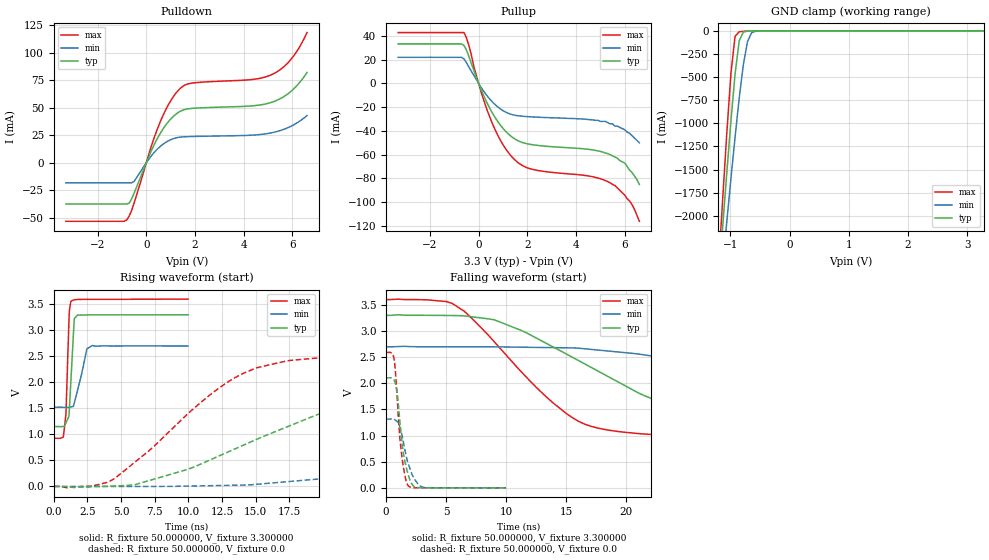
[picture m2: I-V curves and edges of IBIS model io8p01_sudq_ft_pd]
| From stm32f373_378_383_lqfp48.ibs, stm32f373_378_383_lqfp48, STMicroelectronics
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|   Model io8p01_sudq_ft_pd
[Model]  io8p01_sudq_ft_pd
Model_type I/O
Polarity   Non-Inverting
Enable   Active-Low
Vinl =   0.990000V
Vinh =   2.310000V
Vmeas =  1.650000V
Cref =   50.000000pF
Rref =   100.000000M
Vref =   0.0V
C_comp   1.970900pF   1.892300pF   2.063200pF
[Temperature Range]   25.000000   0.125000k   -40.000000
[Pullup Reference]   3.300000V   2.700000V   3.600000V
[Pulldown Reference]   0.0V   0.0V   0.0V
[POWER Clamp Reference]   3.300000V   2.700000V   3.600000V
[GND Clamp Reference]   0.0V   0.0V   0.0V
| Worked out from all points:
|   slope of the pulldown table from 0 to 0.495 V, typ, clamps not added: 20.9 ohm
|   slope of the pullup table from 0 to 0.495 V, typ, clamps not added: 22.2 ohm
|   GND clamp passes 1 mA (typ) near -0.64 V on its own axis
|   rising waveform, R_fixture 50.000000, V_fixture 3.300000: 20-80 % time 269ps typ, 640ps min, 200ps max; typ from 1.15 V to 3.3 V
|   rising waveform, R_fixture 50.000000, V_fixture 0.0: 20-80 % time 12.6ns typ, 30.4ns min, 7.07ns max; typ from 0 V to 2.1 V
|   falling waveform, R_fixture 50.000000, V_fixture 3.300000: 20-80 % time 11ns typ, 22.7ns min, 6.9ns max; typ from 3.3 V to 1.15 V
|   falling waveform, R_fixture 50.000000, V_fixture 0.0: 20-80 % time 664ps typ, 860ps min, 541ps max; typ from 2.1 V to 0 V
[Pulldown]
|Voltage   I(typ)   I(min)   I(max)
-3.3V     -37.45mA   -18.2mA    -53.24mA
-800mV    -37.45mA   -18.2mA    -51.9mA
-700mV    -36.7mA    -18.2mA    -48.48mA
-500mV    -27.71mA   -17.01mA   -36.66mA
200mV     10.57mA    6.084mA    14.57mA
500mV     23.91mA    13.38mA    33.24mA
900mV     37.17mA    19.88mA    52.48mA
1.3V      45.55mA    23.01mA    65.5mA
1.8V      49.29mA    23.83mA    72.18mA
5.1V      54.68mA    27.07mA    79.72mA
5.9V      64.2mA     32.82mA    93.01mA
6.6V      82.13mA    42.97mA    118.5mA
[Pullup]
|Voltage   I(typ)   I(min)   I(max)
-3.3V     33.17mA    21.9mA     42.7mA
-600mV    31.87mA    20.58mA    42.7mA
-400mV    22.79mA    13.76mA    31.9mA
100mV     -5.13mA    -3.299mA   -6.952mA
500mV     -22.5mA    -14.16mA   -30.52mA
900mV     -35.28mA   -21.55mA   -48mA
1.4V      -45.55mA   -26.41mA   -62.54mA
2.2V      -51.57mA   -28.22mA   -72.25mA
5.3V      -59.1mA    -33mA      -82.6mA
6V        -67mA      -39mA      -94mA
6.2V      -73mA      -42mA      -99mA
6.6V      -85mA      -50mA      -116mA
[GND_clamp]
|Voltage   I(typ)   I(min)   I(max)
-3.3V     -9.525A    -9.501A    -9.513A
-1.2V     -2.719A    -3.023A    -2.568A
-1.13V    -2.122A    -2.541A    -1.826A
-1.06V    -1.537A    -2.065A    -1.111A
-990mV    -975.7mA   -1.599A    -462mA
-920mV    -467.5mA   -1.149A    -59.02mA
-850mV    -106.6mA   -727.3mA   -10.13mA
-780mV    -13.08mA   -365.4mA   -5.271mA
-710mV    -3.06mA    -114.8mA   -2.651mA
-640mV    -957.2uA   -20.17mA   -921.6uA
-570mV    -212.9uA   -3.969mA   -172uA
3.28V     83.81uA    63.75uA    93.54uA
[POWER_clamp]
|Voltage   I(typ)   I(min)   I(max)
-3.28V    0A         0A         0A
0V        0A         0A         0A
[Ramp]
| variable   typ   min   max
dV/dt_r  1.26156/12.54362n   0.78870/30.38144n   1.55370/7.05539n
dV/dt_f  1.28928/10.94568n   0.70680/22.67171n   1.60430/6.89156n
R_load = 50.000000
[Rising Waveform]
R_fixture= 50.000000
V_fixture= 3.300000
V_fixture_min= 2.700000
V_fixture_max= 3.600000
|time   V(typ)   V(min)   V(max)
0s        1.15V      1.52V      925.1mV
720.7ps   1.152V     1.52V      978.8mV
900.9ps   1.221V     1.519V     1.392V
1.141ns   1.421V     1.522V     3.31V
1.261ns   1.999V     1.527V     3.552V
1.522ns   3.227V     1.604V     3.586V
1.762ns   3.293V     1.85V      3.592V
2.462ns   3.296V     2.645V     3.594V
2.863ns   3.297V     2.708V     3.595V
9.97ns    3.299V     2.699V     3.599V
[Rising Waveform]
R_fixture= 50.000000
V_fixture= 0.0
V_fixture_min= 0.0
V_fixture_max= 0.0
|time   V(typ)   V(min)   V(max)
0s        1.98nV     11.35nV    2.495nV
4.505ns   8.245mV    25.84uV    149.8mV
10.01ns   333.1mV    6.62mV     1.412V
14.01ns   784.8mV    26.04mV    2.166V
17.52ns   1.165V     95.18mV    2.421V
22.02ns   1.586V     194.8mV    2.524V
32.03ns   1.987V     468.3mV    2.582V
55.56ns   2.099V     1.053V     2.59V
75.08ns   2.102V     1.238V     2.59V
249.2ns   2.102V     1.315V     2.59V
[Falling Waveform]
R_fixture= 50.000000
V_fixture= 3.300000
V_fixture_min= 2.700000
V_fixture_max= 3.600000
|time   V(typ)   V(min)   V(max)
0s        3.299V     2.699V     3.599V
5.506ns   3.296V     2.699V     3.527V
9.009ns   3.215V     2.697V     2.794V
13.51ns   2.743V     2.683V     1.704V
16.52ns   2.374V     2.661V     1.221V
24.52ns   1.517V     2.439V     989.5mV
32.53ns   1.278V     2.152V     947.7mV
42.04ns   1.2V       1.835V     933.5mV
70.57ns   1.156V     1.581V     925mV
249.2ns   1.15V      1.52V      925.1mV
[Falling Waveform]
R_fixture= 50.000000
V_fixture= 0.0
V_fixture_min= 0.0
V_fixture_max= 0.0
|time   V(typ)   V(min)   V(max)
0s        2.102V     1.315V     2.59V
660.7ps   2.06V      1.314V     2.464V
900.9ps   1.839V     1.271V     1.793V
1.141ns   1.272V     1.163V     949.5mV
1.261ns   974.3mV    1.073V     691.1mV
1.602ns   461.9mV    684.2mV    189.4mV
1.862ns   235.9mV    450.5mV    34.15mV
2.282ns   33.01mV    202.5mV    4.353mV
3.103ns   1.374mV    10.53mV    452.6uV
9.97ns    1.98nV     11.35nV    2.495nV
